TYPE STR_CDG200D :
STRUCT
	Reading_Valid1					:BOOL;
	Overrange_Exceeded1				:BOOL;
	Underrange_Exceeded1			:BOOL;
	Sensor_Value1					:REAL;
	Reading_Valid2					:BOOL;
	Overrange_Exceeded2				:BOOL;
	Underrange_Exceeded2			:BOOL;
	Sensor_Value2					:REAL;
	Active_Exception_Status			:USINT;
	Trip_Point_Output_All_Insta		:UDINT;
END_STRUCT
END_TYPE
